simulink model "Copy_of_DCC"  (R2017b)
settings: Solver=FixedStepDiscrete  StartTime=0.0  StopTime=10.0  FixedStep=0.01  RelTol=1e-3  EnableMultiTasking=on
undefined symbols (not defined in the file): ASWTYPE_FALSE, ASWTYPE_TRUE, CbDCC_BMTMsgCmd_flg, CbDCC_BMVMsgCmd_flg, CbDCC_BSPMsgCmd_flg, CcDCC_BSTSendTi_ms, CcDCC_BulkSOC_pct, CcDCC_CCSTout_ms, CcDCC_CellTempFilterAvg_numb, CcDCC_ChrgCrnt0HysVolt_mV, CcDCC_ChrgFinOverTi_ms, CcDCC_ChrgMaxPackVoltLimt_V, CcDCC_ChrgSt2StepChrgTime_ms, CcDCC_ChrgStCutoffTime_ms, CcDCC_ChrgStFullChrgCrnt_A, CcDCC_CMLTout_ms, CcDCC_CommToutOverTi_ms, CcDCC_CRMAATout_ms, CcDCC_CRMCHMTout_ms, CcDCC_CRMTout_ms, CcDCC_CROAATout_ms, CcDCC_CROTout_ms, CcDCC_CSDTout_ms, CcDCC_CSTTout_ms, CcDCC_DC12VUnonnectTi_ms, CcDCC_DCChrgDispSOCPrmt_pct, CcDCC_DCChrgMismatch_ms, CcDCC_DCChrgPermitCfg_ms, CcDCC_DCChrgPrmtFltLvl_numb, CcDCC_DCChrgPrmtStop_ms, CcDCC_DCChrgStepCurr_A, CcDCC_DCChrgStop_ms, CcDCC_DCCrntUnctrolTi_ms, CcDCC_DCFullChrgHysVolt_mV, CcDCC_DCFullStepChrgTi1_ms, CcDCC_DCFullStepChrgTi2_ms, CcDCC_DCMaxChrgCurr_A, CcDCC_DCStepChrgWaitTime_ms, CcDCC_DCStop2DefaultTi_ms, CcDCC_DefaultWaitTi_ms, CcDCC_DiffDCChrgCrnt_A, CcDCC_DiffDCChrgCrntTi_ms, CcDCC_HeatChrgCrnt0Time_ms, CcDCC_HeatChrgCrnt1Time_ms, CcDCC_IsoDisableDelay_ms, CcDCC_MaxPackVoltLimt_V, CcDCC_SafeCur_A, CcDCC_StartChrgHysVolt_mV, CcDCC_StartDCChrgCellTemp_C, CcDCC_StepChrgCutoffTi_ms, CcDCC_StepChrgFullChrgCrnt_A, CcDCC_ToutDelay_ms, CcDCC_VehSpdFld_kmh, DCC_CONST0_NUMB, DCC_CONST1000_NUMB, DCC_CONST170_NUMB, DCC_RUNTIME_MS, Enum_BTMHeatReq, Enum_CTCCtrCtlConnMode, Enum_CTCCtrCtlState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
libraries: AIWAYS_Powertrain_BMS_lib x82
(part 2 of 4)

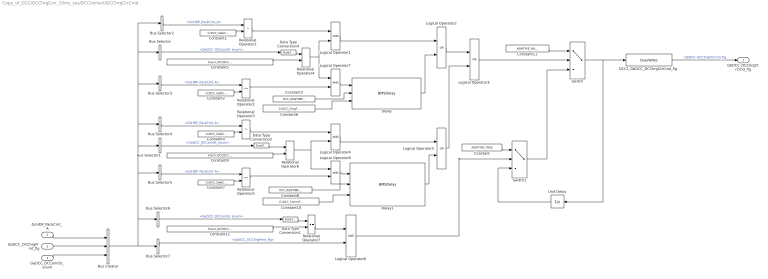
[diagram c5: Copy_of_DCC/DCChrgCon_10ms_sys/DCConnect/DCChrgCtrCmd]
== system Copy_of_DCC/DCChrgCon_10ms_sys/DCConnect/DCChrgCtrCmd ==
  GcHDP_PackCrnt_A : Inport
  GbDCC_DCChrgPrmt_flg : Inport  Port=2
  GeDCC_DCConnSt_enum : Inport  Port=3
  Bus Creator : BusCreator  Inputs=3
  Bus Selector : BusSelector  OutputSignals=GeDCC_DCConnSt_enum
  Bus Selector1 : BusSelector  OutputSignals=GeDCC_DCConnSt_enum
  Bus Selector{2..5} (4 alike) : BusSelector  OutputSignals=GcHDP_PackCrnt_A
  Bus Selector6 : BusSelector  OutputSignals=GeDCC_DCConnSt_enum
  Bus Selector7 : BusSelector  OutputSignals=GbDCC_DCChrgPrmt_flg
  Constant : Constant  Value=ASWTYPE_TRUE
  Constant{1..2,4,7} (4 alike) : Constant  Value=CcDCC_SafeCur_A
  Constant10 : Constant  Value=CcDCC_CommToutOverTi_ms
  Constant11 : Constant  Value=ASWTYPE_FALSE
  Constant12 : Constant  Value=Enum_DCCDCConnSt.Enum_DCCDCConnSt_CFG
  Constant3 : Constant  Value=DCC_RUNTIME_MS
  Constant5 : Constant  Value=Enum_DCCDCConnSt.Enum_DCCDCConnSt_ChrgFin
  Constant6 : Constant  Value=CcDCC_ChrgFinOverTi_ms
  Constant8 : Constant  Value=DCC_RUNTIME_MS
  Constant9 : Constant  Value=Enum_DCCDCConnSt.Enum_DCCDCConnSt_CommTout
  DCC1_GbDCC_DCChrgCtrCmd_flg : AIWAYS_Powertrain_BMS_lib/Signals/OverWrite  OverWrite_Value=CbDCC_DCChrgCtrCmdOvr_flg  OverWrite_flag=CbDCC_DCChrgCtrCmdOvrSwt_flg
  Data Type Conversion1 : DataTypeConversion
  Data Type Conversion2 : DataTypeConversion
  Data Type Conversion4 : DataTypeConversion
  Delay : AIWAYS_Powertrain_BMS_lib/Debounce & Delay/BMSDelay
  Delay1 : AIWAYS_Powertrain_BMS_lib/Debounce & Delay/BMSDelay
  Logical Operator{1,4,6..8} (5 alike) : Logic  AllPortsSameDT=off  OutDataTypeStr=boolean
  Logical Operator2 : Logic  Operator=OR  AllPortsSameDT=off  OutDataTypeStr=boolean
  Logical Operator3 : Logic  Operator=OR  AllPortsSameDT=off  OutDataTypeStr=boolean
  Logical Operator5 : Logic  Operator=OR  AllPortsSameDT=off  OutDataTypeStr=boolean
  Relational Operator1 : RelationalOperator  Operator=>  OutDataTypeStr=boolean
  Relational Operator2 : RelationalOperator  Operator=<=  OutDataTypeStr=boolean
  Relational Operator3 : RelationalOperator  Operator=>  OutDataTypeStr=boolean
  Relational Operator4 : RelationalOperator  Operator===  OutDataTypeStr=boolean
  Relational Operator5 : RelationalOperator  Operator=<=  OutDataTypeStr=boolean
  Relational Operator6 : RelationalOperator  Operator===  OutDataTypeStr=boolean
  Relational Operator7 : RelationalOperator  Operator===  OutDataTypeStr=boolean
  Switch : Switch  Criteria=u2 ~= 0
  Switch1 : Switch  Criteria=u2 ~= 0
  Unit Delay : UnitDelay  SampleTime=-1  StateName=StateName
  GbDCC_DCChrgCtrCmd_flg : Outport
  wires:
  Constant2/1 -> Relational Operator2/2
  Bus Selector7/1 -> Logical Operator6/2  "<GbDCC_DCChrgPrmt_flg>"
  Switch/1 -> DCC1_GbDCC_DCChrgCtrCmd_flg/1, Unit Delay/1
  Bus Selector6/1 -> Data Type Conversion1/1  "<GeDCC_DCConnSt_enum>"
  Constant12/1 -> Relational Operator7/2
  Relational Operator7/1 -> Logical Operator6/1
  Constant3/1 -> Delay/2
  Switch1/1 -> Switch/3
  Unit Delay/1 -> Switch1/3
  Logical Operator3/1 -> Switch/2
  Constant11/1 -> Switch/1
  Constant/1 -> Switch1/1
  Constant6/1 -> Delay/3
  Constant1/1 -> Relational Operator1/2
  Constant10/1 -> Delay1/3
  Constant7/1 -> Relational Operator5/2
  Constant9/1 -> Relational Operator6/2
  Constant4/1 -> Relational Operator3/2
  Constant8/1 -> Delay1/2
  Constant5/1 -> Relational Operator4/2
  Logical Operator6/1 -> Switch1/2
  Bus Selector2/1 -> Relational Operator1/1  "<GcHDP_PackCrnt_A>"
  Bus Selector/1 -> Data Type Conversion4/1  "<GeDCC_DCConnSt_enum>"
  Bus Selector1/1 -> Data Type Conversion2/1  "<GeDCC_DCConnSt_enum>"
  Bus Selector4/1 -> Relational Operator3/1  "<GcHDP_PackCrnt_A>"
  Bus Selector3/1 -> Relational Operator2/1  "<GcHDP_PackCrnt_A>"
  Bus Creator/1 -> Bus Selector2/1, Bus Selector/1, Bus Selector3/1, Bus Selector4/1, Bus Selector1/1, Bus Selector5/1, Bus Selector6/1, Bus Selector7/1
  Bus Selector5/1 -> Relational Operator5/1  "<GcHDP_PackCrnt_A>"
  DCC1_GbDCC_DCChrgCtrCmd_flg/1 -> GbDCC_DCChrgCtrCmd_flg/1  "GbDCC_DCChrgCtrCmd_flg"
  Data Type Conversion4/1 -> Relational Operator4/1
  Data Type Conversion2/1 -> Relational Operator6/1
  Data Type Conversion1/1 -> Relational Operator7/1
  Logical Operator1/1 -> Logical Operator2/1
  Relational Operator1/1 -> Logical Operator1/1
  Relational Operator4/1 -> Logical Operator7/1, Logical Operator1/2
  Relational Operator2/1 -> Logical Operator7/2
  Logical Operator7/1 -> Delay/1
  Delay/1 -> Logical Operator2/2
  Logical Operator2/1 -> Logical Operator3/1
  Logical Operator5/1 -> Logical Operator3/2
  Relational Operator6/1 -> Logical Operator8/1, Logical Operator4/2
  Relational Operator3/1 -> Logical Operator4/1
  Logical Operator4/1 -> Logical Operator5/1
  Relational Operator5/1 -> Logical Operator8/2
  Logical Operator8/1 -> Delay1/1
  Delay1/1 -> Logical Operator5/2
  GcHDP_PackCrnt_A/1 -> Bus Creator/1
  GbDCC_DCChrgPrmt_flg/1 -> Bus Creator/2
  GeDCC_DCConnSt_enum/1 -> Bus Creator/3

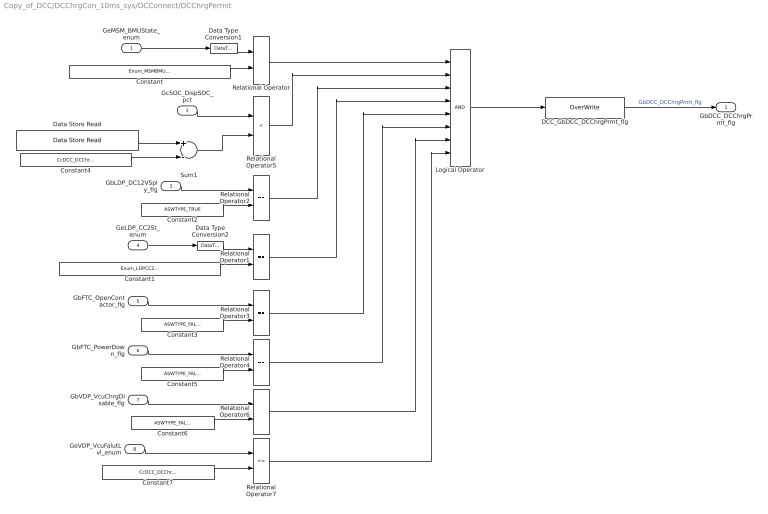
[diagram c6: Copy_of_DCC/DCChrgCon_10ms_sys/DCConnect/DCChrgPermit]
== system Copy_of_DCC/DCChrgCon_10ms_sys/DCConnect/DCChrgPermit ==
  GeMSM_BMUState_enum : Inport
  GcSOC_DispSOC_pct : Inport  Port=2
  GbLDP_DC12VSply_flg : Inport  Port=3
  GeLDP_CC2St_enum : Inport  Port=4
  GbFTC_OpenContactor_flg : Inport  Port=5
  GbFTC_PowerDown_flg : Inport  Port=6
  GbVDP_VcuChrgDisable_flg : Inport  Port=7
  GeVDP_VcuFalutLvl_enum : Inport  Port=8
  Constant : Constant  Value=Enum_MSMBMUState.Enum_MSMBMUState_Run
  Constant1 : Constant  Value=Enum_LDPCC2St.Enum_LDPCC2St_Connect
  Constant2 : Constant  Value=ASWTYPE_TRUE
  Constant3 : Constant  Value=ASWTYPE_FALSE
  Constant4 : Constant  Value=CcDCC_DCChrgDispSOCPrmt_pct
  Constant5 : Constant  Value=ASWTYPE_FALSE
  Constant6 : Constant  Value=ASWTYPE_FALSE
  Constant7 : Constant  Value=CcDCC_DCChrgPrmtFltLvl_numb
  DCC_GbDCC_DCChrgPrmt_flg : AIWAYS_Powertrain_BMS_lib/Signals/OverWrite  OverWrite_Value=CbDCC_DCChrgPrmtOvr_flg  OverWrite_flag=CbDCC_DCChrgPrmtOvrSwt_flg
  Data Store Read : AIWAYS_Powertrain_BMS_lib/Signals/Data Store Read  Priority=0  DSR=EcNVM_ChrgPermitMaxSOC_pct
  Data Type Conversion1 : DataTypeConversion
  Data Type Conversion2 : DataTypeConversion
  Logical Operator : Logic  Inputs=8  AllPortsSameDT=off  OutDataTypeStr=boolean
  Relational Operator{,1..4,6} (6 alike) : RelationalOperator  Operator===  OutDataTypeStr=boolean
  Relational Operator5 : RelationalOperator  Operator=<  OutDataTypeStr=boolean
  Relational Operator7 : RelationalOperator  Operator=<=  OutDataTypeStr=boolean
  Sum1 : Sum  Inputs=+-  OutDataTypeStr=Inherit: Inherit via back propagation  RndMeth=Zero
  GbDCC_DCChrgPrmt_flg : Outport
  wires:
  Constant/1 -> Relational Operator/2
  GeMSM_BMUState_enum/1 -> Data Type Conversion1/1
  Logical Operator/1 -> DCC_GbDCC_DCChrgPrmt_flg/1
  GbLDP_DC12VSply_flg/1 -> Relational Operator2/1
  GeLDP_CC2St_enum/1 -> Data Type Conversion2/1
  Constant1/1 -> Relational Operator1/2
  Data Type Conversion1/1 -> Relational Operator/1
  GcSOC_DispSOC_pct/1 -> Relational Operator5/1
  Constant2/1 -> Relational Operator2/2
  Relational Operator/1 -> Logical Operator/1
  DCC_GbDCC_DCChrgPrmt_flg/1 -> GbDCC_DCChrgPrmt_flg/1  "GbDCC_DCChrgPrmt_flg"
  Data Type Conversion2/1 -> Relational Operator1/1
  Relational Operator2/1 -> Logical Operator/3
  Relational Operator1/1 -> Logical Operator/4
  Constant3/1 -> Relational Operator3/2
  GbFTC_OpenContactor_flg/1 -> Relational Operator3/1
  Constant5/1 -> Relational Operator4/2
  GbFTC_PowerDown_flg/1 -> Relational Operator4/1
  Constant6/1 -> Relational Operator6/2
  GbVDP_VcuChrgDisable_flg/1 -> Relational Operator6/1
  Relational Operator3/1 -> Logical Operator/5
  Relational Operator4/1 -> Logical Operator/6
  Relational Operator6/1 -> Logical Operator/7
  GeVDP_VcuFalutLvl_enum/1 -> Relational Operator7/1
  Constant7/1 -> Relational Operator7/2
  Relational Operator7/1 -> Logical Operator/8
  Relational Operator5/1 -> Logical Operator/2
  Data Store Read/1 -> Sum1/1
  Constant4/1 -> Sum1/2
  Sum1/1 -> Relational Operator5/2

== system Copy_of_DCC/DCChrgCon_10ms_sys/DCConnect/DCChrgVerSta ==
  Constant2 : Constant  Value=ASWTYPE_TRUE
  DCC1_GbDCC_DCChrgVerSta_flg : AIWAYS_Powertrain_BMS_lib/Signals/OverWrite  OverWrite_Value=CbDCC_DCChrgVerStaOvr_flg  OverWrite_flag=CbDCC_DCChrgVerStaOvrSwt_flg
  GbDCC_DCChrgVerSta_flg : Outport
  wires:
  DCC1_GbDCC_DCChrgVerSta_flg/1 -> GbDCC_DCChrgVerSta_flg/1  "GbDCC_DCChrgVerSta_flg"
  Constant2/1 -> DCC1_GbDCC_DCChrgVerSta_flg/1

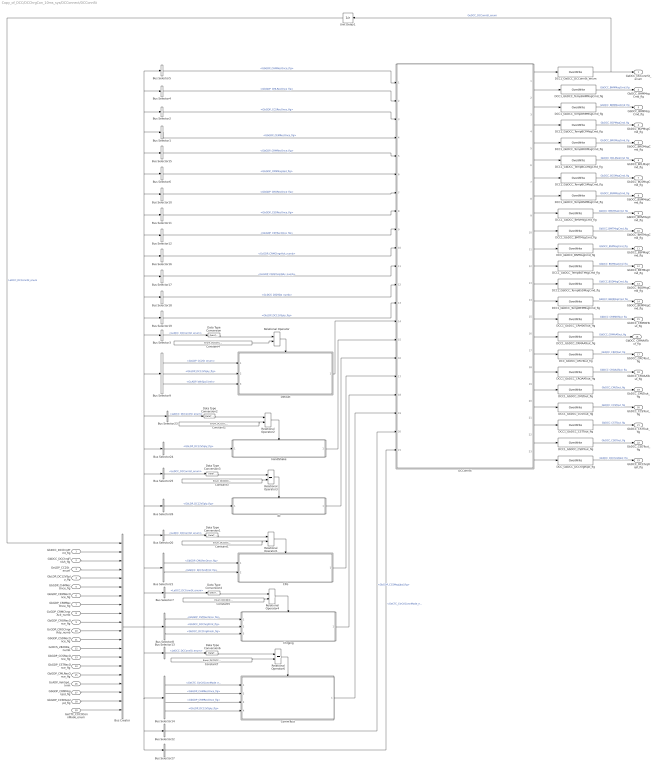
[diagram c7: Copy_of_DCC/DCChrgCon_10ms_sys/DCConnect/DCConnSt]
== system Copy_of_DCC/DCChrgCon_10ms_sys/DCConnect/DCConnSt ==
  GbDCC_DCChrgPrmt_flg : Inport
  GbDCC_DCChrgFinish_flg : Inport  Port=2
  GeLDP_CC2St_enum : Inport  Port=3
  GbLDP_DC12VSply_flg : Inport  Port=4
  GbGDP_CHMRecOnce_flg : Inport  Port=5
  GbGDP_CEMRecOnce_flg : Inport  Port=6
  GbGDP_CRMRecOnce_flg : Inport  Port=7
  GcGDP_CRMChrgrAck_numb : Inport  Port=8
  GbGDP_CRORecOnce_flg : Inport  Port=9
  GcGDP_CROChrgrRdy_numb : Inport  Port=10
  GbGDP_CSDRecOnce_flg : Inport  Port=11
  GcDCS_2829Da_numb : Inport  Port=12
  GbGDP_CCSRecOnce_flg : Inport  Port=13
  GbGDP_CSTRecOnce_flg : Inport  Port=14
  GbGDP_CMLRecOnce_flg : Inport  Port=15
  GcADP_VehSpd_kmh : Inport  Port=16
  GbGDP_CRMMsgUpd_flg : Inport  Port=17
  GbGDP_CCSMsgUpd_flg : Inport  Port=18
  GeCTC_CtrCtlConnMode_enum : Inport  Port=19
  Bus Creator : BusCreator  Inputs=20
  Bus Selector1 : BusSelector  OutputSignals=GbGDP_CEMRecOnce_flg
  Bus Selector10 : BusSelector  OutputSignals=GbGDP_CRORecOnce_flg
  Bus Selector11 : BusSelector  OutputSignals=GbGDP_CSDRecOnce_flg
  Bus Selector12 : BusSelector  OutputSignals=GbGDP_CSTRecOnce_flg
  Bus Selector{3,7,13,20,23,25} (6 alike) : BusSelector  OutputSignals=LeDCC_DCConnSt_enum
  Bus Selector14 : BusSelector  OutputSignals=GeCTC_CtrCtlConnMode_enum,GbGDP_CHMRecOnce_flg,GbGDP_CRMRecOnce_flg,GbLDP_DC12VSply_flg
  Bus Selector15 : BusSelector  OutputSignals=GbGDP_CRMRecOnce_flg
  Bus Selector16 : BusSelector  OutputSignals=GcGDP_CRMChrgrAck_numb
  Bus Selector17 : BusSelector  OutputSignals=GcGDP_CROChrgrRdy_numb
  Bus Selector18 : BusSelector  OutputSignals=GcDCS_2829Da_numb
  Bus Selector19 : BusSelector  OutputSignals=GbLDP_DC12VSply_flg
  Bus Selector2 : BusSelector  OutputSignals=GbGDP_CCSRecOnce_flg
  Bus Selector21 : BusSelector  OutputSignals=GbGDP_CMLRecOnce_flg,GbDCC_DCChrgPrmt_flg
  Bus Selector22 : BusSelector  OutputSignals=GbGDP_CCSMsgUpd_flg
  Bus Selector24 : BusSelector  OutputSignals=GbLDP_DC12VSply_flg
  Bus Selector26 : BusSelector  OutputSignals=GbLDP_DC12VSply_flg
  Bus Selector27 : BusSelector  OutputSignals=GeCTC_CtrCtlConnMode_enum
  Bus Selector4 : BusSelector  OutputSignals=GbGDP_CMLRecOnce_flg
  Bus Selector5 : BusSelector  OutputSignals=GbGDP_CHMRecOnce_flg
  Bus Selector6 : BusSelector  OutputSignals=GbGDP_CRMMsgUpd_flg
  Bus Selector8 : BusSelector  OutputSignals=GbGDP_CSTRecOnce_flg,GbDCC_DCChrgPrmt_flg,GbDCC_DCChrgFinish_flg
  Bus Selector9 : BusSelector  OutputSignals=GeLDP_CC2St_enum,GbLDP_DC12VSply_flg,GcADP_VehSpd_kmh
  CFG : Subsystem
  Chrging : Subsystem
  CommTout : Subsystem
  Constant1 : Constant  Value=Enum_DCCDCConnSt.Enum_DCCDCConnSt_CFG
  Constant2 : Constant  Value=Enum_DCCDCConnSt.Enum_DCCDCConnSt_HandShake
  Constant3 : Constant  Value=Enum_DCCDCConnSt.Enum_DCCDCConnSt_ID
  Constant4 : Constant  Value=Enum_DCCDCConnSt.Enum_DCCDCConnSt_Default
  Constant5 : Constant  Value=Enum_DCCDCConnSt.Enum_DCCDCConnSt_Chrging
  Constant7 : Constant  Value=Enum_DCCDCConnSt.Enum_DCCDCConnSt_CommTout
  DCC1_GbDCC_BMTMsgCmd_flg : AIWAYS_Powertrain_BMS_lib/Signals/OverWrite  OverWrite_Value=CbDCC_BMTMsgCmdOvr_flg  OverWrite_flag=CbDCC_BMTMsgCmdOvrSwt_flg
  DCC1_GbDCC_BMVMsgCmd_flg : AIWAYS_Powertrain_BMS_lib/Signals/OverWrite  OverWrite_Value=CbDCC_BMVMsgCmdOvr_flg  OverWrite_flag=CbDCC_BMVMsgCmdOvrSwt_flg
  DCC1_GbDCC_CCSTout_flg : AIWAYS_Powertrain_BMS_lib/Signals/OverWrite  OverWrite_Value=CbDCC_CCSToutOvr_flg  OverWrite_flag=CbDCC_CCSToutOvrSwt_flg
  DCC1_GbDCC_CMLTout_flg : AIWAYS_Powertrain_BMS_lib/Signals/OverWrite  OverWrite_Value=CbDCC_CMLToutOvr_flg  OverWrite_flag=CbDCC_CMLToutOvrSwt_flg
  DCC1_GbDCC_CRM00Tout_flg : AIWAYS_Powertrain_BMS_lib/Signals/OverWrite  OverWrite_Value=CbDCC_CRM00ToutOvr_flg  OverWrite_flag=CbDCC_CRM00ToutOvrSwt_flg
  DCC1_GbDCC_CRMAATout_flg : AIWAYS_Powertrain_BMS_lib/Signals/OverWrite  OverWrite_Value=CbDCC_CRMAAToutOvr_flg  OverWrite_flag=CbDCC_CRMAAToutOvrSwt_flg
  DCC1_GbDCC_CROAATout_flg : AIWAYS_Powertrain_BMS_lib/Signals/OverWrite  OverWrite_Value=CbDCC_CROAAToutOvr_flg  OverWrite_flag=CbDCC_CROAAToutOvrSwt_flg
  DCC1_GbDCC_CSDTout_flg : AIWAYS_Powertrain_BMS_lib/Signals/OverWrite  OverWrite_Value=CbDCC_CSDToutOvr_flg  OverWrite_flag=CbDCC_CSDToutOvrSwt_flg
  DCC1_GbDCC_CSTTout_flg : AIWAYS_Powertrain_BMS_lib/Signals/OverWrite  OverWrite_Value=CbDCC_CSTToutOvr_flg  OverWrite_flag=CbDCC_CSTToutOvrSwt_flg
  DCC1_GbDCC_TempBCLMsgCmd_flg : AIWAYS_Powertrain_BMS_lib/Signals/OverWrite  OverWrite_Value=CbDCC_BCLMsgCmdOvr_flg  OverWrite_flag=CbDCC_BCLMsgCmdOvrSwt_flg
  DCC1_GbDCC_TempBCPMsgCmd_flg : AIWAYS_Powertrain_BMS_lib/Signals/OverWrite  OverWrite_Value=CbDCC_BCPMsgCmdOvr_flg  OverWrite_flag=CbDCC_BCPMsgCmdOvrSwt_flg
  DCC1_GbDCC_TempBCSMsgCmd_flg : AIWAYS_Powertrain_BMS_lib/Signals/OverWrite  OverWrite_Value=CbDCC_BCSMsgCmdOvr_flg  OverWrite_flag=CbDCC_BCSMsgCmdOvrSwt_flg
  DCC1_GbDCC_TempBEMMsgCmd_flg : AIWAYS_Powertrain_BMS_lib/Signals/OverWrite  OverWrite_Value=CbDCC_BEMMsgCmdOvr_flg  OverWrite_flag=CbDCC_BEMMsgCmdOvrSwt_flg
  DCC1_GbDCC_TempBHMMsgCmd_flg : AIWAYS_Powertrain_BMS_lib/Signals/OverWrite  OverWrite_Value=CbDCC_BHMMsgCmdOvr_flg  OverWrite_flag=CbDCC_BHMMsgCmdOvrSwt_flg
  DCC1_GbDCC_TempBRMMsgCmd_flg : AIWAYS_Powertrain_BMS_lib/Signals/OverWrite  OverWrite_Value=CbDCC_BRMMsgCmdOvr_flg  OverWrite_flag=CbDCC_BRMMsgCmdOvrSwt_flg
  DCC1_GbDCC_TempBROMsgCmd_flg : AIWAYS_Powertrain_BMS_lib/Signals/OverWrite  OverWrite_Value=CbDCC_BROMsgCmdOvr_flg  OverWrite_flag=CbDCC_BROMsgCmdOvrSwt_flg
  DCC1_GbDCC_TempBSDMsgCmd_flg : AIWAYS_Powertrain_BMS_lib/Signals/OverWrite  OverWrite_Value=CbDCC_BSDMsgCmdOvr_flg  OverWrite_flag=CbDCC_BSDMsgCmdOvrSwt_flg
  DCC1_GbDCC_TempBSMMsgCmd_flg : AIWAYS_Powertrain_BMS_lib/Signals/OverWrite  OverWrite_Value=CbDCC_BSMMsgCmdOvr_flg  OverWrite_flag=CbDCC_BSMMsgCmdOvrSwt_flg
  DCC1_GbDCC_TempBSTMsgCmd_flg : AIWAYS_Powertrain_BMS_lib/Signals/OverWrite  OverWrite_Value=CbDCC_BSTMsgCmdOvr_flg  OverWrite_flag=CbDCC_BSTMsgCmdOvrSwt_flg
  DCC1_GeDCC_DCConnSt_enum : AIWAYS_Powertrain_BMS_lib/Signals/OverWrite  OverWrite_Value=CeDCC_DCConnStOvr_enum  OverWrite_flag=CbDCC_DCConnStOvrSwt_flg
  DCC_GbDCC_BSPMsgCmd_flg : AIWAYS_Powertrain_BMS_lib/Signals/OverWrite  OverWrite_Value=CbDCC_BSPMsgCmdOvr_flg  OverWrite_flag=CbDCC_BSPMsgCmdOvrSwt_flg
  DCC_GbDCC_CROTout_flg : AIWAYS_Powertrain_BMS_lib/Signals/OverWrite  OverWrite_Value=CbDCC_CROToutOvr_flg  OverWrite_flag=CbDCC_CROToutOvrSwt_flg
  DCC_GbDCC_DCChrgRqst_flg : AIWAYS_Powertrain_BMS_lib/Signals/OverWrite  OverWrite_Value=CbDCC_DCChrgRqstOvr_flg  OverWrite_flag=CbDCC_DCChrgRqstOvrSwt_flg
  DCConnSt : Stateflow chart  TreatAsAtomicUnit=on
  Data Type Conversion{,1..4,6} (6 alike) : DataTypeConversion
  Default : Subsystem
  HandShake : Subsystem
  ID : Subsystem
  Relational Operator{,1..4,6} (6 alike) : RelationalOperator  Operator===  OutDataTypeStr=boolean
  Unit Delay1 : UnitDelay  SampleTime=-1  StateName=StateName
  GeDCC_DCConnSt_enum : Outport
  GbDCC_BHMMsgCmd_flg : Outport  Port=2
  GbDCC_BRMMsgCmd_flg : Outport  Port=3
  GbDCC_BCPMsgCmd_flg : Outport  Port=4
  GbDCC_BROMsgCmd_flg : Outport  Port=5
  GbDCC_BCLMsgCmd_flg : Outport  Port=6
  GbDCC_BCSMsgCmd_flg : Outport  Port=7
  GbDCC_BSMMsgCmd_flg : Outport  Port=8
  GbDCC_BMVMsgCmd_flg : Outport  Port=9
  GbDCC_BMTMsgCmd_flg : Outport  Port=10
  GbDCC_BSPMsgCmd_flg : Outport  Port=11
  GbDCC_BSTMsgCmd_flg : Outport  Port=12
  GbDCC_BSDMsgCmd_flg : Outport  Port=13
  GbDCC_BEMMsgCmd_flg : Outport  Port=14
  GbDCC_CRM00Tout_flg : Outport  Port=15
  GbDCC_CRMAATout_flg : Outport  Port=16
  GbDCC_CROTout_flg : Outport  Port=17
  GbDCC_CROAATout_flg : Outport  Port=18
  GbDCC_CMLTout_flg : Outport  Port=19
  GbDCC_CCSTout_flg : Outport  Port=20
  GbDCC_CSTTout_flg : Outport  Port=21
  GbDCC_CSDTout_flg : Outport  Port=22
  GbDCC_DCChrgRqst_flg : Outport  Port=23
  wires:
  Bus Selector19/1 -> DCConnSt/13(GbLDP_DC12VSply_flg)  "<GbLDP_DC12VSply_flg>"
  Bus Selector18/1 -> DCConnSt/12(GcDCS_2829Da_numb)  "<GcDCS_2829Da_numb>"
  Bus Selector17/1 -> DCConnSt/11(GcGDP_CROChrgrRdy_numb)  "<GcGDP_CROChrgrRdy_numb>"
  Bus Selector16/1 -> DCConnSt/10(GcGDP_CRMChrgrAck_numb)  "<GcGDP_CRMChrgrAck_numb>"
  Bus Selector12/1 -> DCConnSt/9(GbGDP_CSTRecOnce_flg)  "<GbGDP_CSTRecOnce_flg>"
  Bus Selector11/1 -> DCConnSt/8(GbGDP_CSDRecOnce_flg)  "<GbGDP_CSDRecOnce_flg>"
  Bus Selector10/1 -> DCConnSt/7(GbGDP_CRORecOnce_flg)  "<GbGDP_CRORecOnce_flg>"
  Bus Selector6/1 -> DCConnSt/6(GbGDP_CRMMsgUpd_flg)  "<GbGDP_CRMMsgUpd_flg>"
  Bus Selector5/1 -> DCConnSt/1(GbGDP_CHMRecOnce_flg)  "<GbGDP_CHMRecOnce_flg>"
  Bus Selector4/1 -> DCConnSt/2(GbGDP_CMLRecOnce_flg)  "<GbGDP_CMLRecOnce_flg>"
  Bus Selector2/1 -> DCConnSt/3(GbGDP_CCSRecOnce_flg)  "<GbGDP_CCSRecOnce_flg>"
  Bus Selector1/1 -> DCConnSt/4(GbGDP_CEMRecOnce_flg)  "<GbGDP_CEMRecOnce_flg>"
  DCConnSt/22(GbDCC_CSDTout_flg) -> DCC1_GbDCC_CSDTout_flg/1
  DCConnSt/21(GbDCC_CSTTout_flg) -> DCC1_GbDCC_CSTTout_flg/1
  DCConnSt/20(GbDCC_CCSTout_flg) -> DCC1_GbDCC_CCSTout_flg/1
  DCConnSt/19(GbDCC_CMLTout_flg) -> DCC1_GbDCC_CMLTout_flg/1
  DCConnSt/18(GbDCC_CROAATout_flg) -> DCC1_GbDCC_CROAATout_flg/1
  DCConnSt/17(GbDCC_CROTout_flg) -> DCC_GbDCC_CROTout_flg/1
  DCConnSt/16(GbDCC_CRMAATout_flg) -> DCC1_GbDCC_CRMAATout_flg/1
  DCC1_GbDCC_CSDTout_flg/1 -> GbDCC_CSDTout_flg/1  "GbDCC_CSDTout_flg"
  DCC1_GbDCC_CSTTout_flg/1 -> GbDCC_CSTTout_flg/1  "GbDCC_CSTTout_flg"
  DCC1_GbDCC_CCSTout_flg/1 -> GbDCC_CCSTout_flg/1  "GbDCC_CCSTout_flg"
  DCC_GbDCC_CROTout_flg/1 -> GbDCC_CROTout_flg/1  "GbDCC_CROTout_flg"
  DCC1_GbDCC_CROAATout_flg/1 -> GbDCC_CROAATout_flg/1  "GbDCC_CROAATout_flg"
  DCC1_GbDCC_CMLTout_flg/1 -> GbDCC_CMLTout_flg/1  "GbDCC_CMLTout_flg"
  DCC1_GbDCC_CRMAATout_flg/1 -> GbDCC_CRMAATout_flg/1  "GbDCC_CRMAATout_flg"
  DCC1_GbDCC_CRM00Tout_flg/1 -> GbDCC_CRM00Tout_flg/1  "GbDCC_CRM00Tout_flg"
  DCConnSt/15(GbDCC_CRM00Tout_flg) -> DCC1_GbDCC_CRM00Tout_flg/1
  Bus Selector15/1 -> DCConnSt/5(GbGDP_CRMRecOnce_flg)  "<GbGDP_CRMRecOnce_flg>"
  Unit Delay1/1 -> Bus Creator/1  "LeDCC_DCConnSt_enum"
  Data Type Conversion6/1 -> Relational Operator6/1
  Data Type Conversion4/1 -> Relational Operator4/1
  Data Type Conversion/1 -> Relational Operator/1
  DCConnSt/1(GeDCC_DCConnSt_enum) -> DCC1_GeDCC_DCConnSt_enum/1
  Bus Selector9/3 -> Default/3(GcADP_VehSpd_kmh)  "<GcADP_VehSpd_kmh>"
  Chrging/1(LbDCC_DCChrging2ChrgFin_flg) -> DCConnSt/18(LbDCC_DCChrging2ChrgFin_flg)
  CommTout/1(LbDCC_DCCommTout2Default_flg) -> DCConnSt/19(LbDCC_DCCommTout2Default_flg)
  Default/1(LbDCC_DCDefault2Handshake_flg) -> DCConnSt/14(LbDCC_DCDefault2Handshake_flg)
  DCC1_GbDCC_BMVMsgCmd_flg/1 -> GbDCC_BMVMsgCmd_flg/1  "GbDCC_BMVMsgCmd_flg"
  DCC1_GbDCC_BMTMsgCmd_flg/1 -> GbDCC_BMTMsgCmd_flg/1  "GbDCC_BMTMsgCmd_flg"
  DCC_GbDCC_BSPMsgCmd_flg/1 -> GbDCC_BSPMsgCmd_flg/1  "GbDCC_BSPMsgCmd_flg"
  DCC1_GeDCC_DCConnSt_enum/1 -> GeDCC_DCConnSt_enum/1, Unit Delay1/1  "GeDCC_DCConnSt_enum"
  Bus Selector14/1 -> CommTout/1(GeCTC_CtrCtlConnMode_enum)  "<GeCTC_CtrCtlConnMode_enum>"
  Bus Selector13/1 -> Data Type Conversion6/1  "<LeDCC_DCConnSt_enum>"
  Bus Selector8/3 -> Chrging/3(GbDCC_DCChrgFinish_flg)  "<GbDCC_DCChrgFinish_flg>"
  Bus Selector8/2 -> Chrging/2(GbDCC_DCChrgPrmt_flg)  "<GbDCC_DCChrgPrmt_flg>"
  Bus Selector8/1 -> Chrging/1(GbGDP_CSTRecOnce_flg)  "<GbGDP_CSTRecOnce_flg>"
  Bus Selector9/2 -> Default/2(GbLDP_DC12VSply_flg)  "<GbLDP_DC12VSply_flg>"
  Bus Selector9/1 -> Default/1(GeLDP_CC2St_enum)  "<GeLDP_CC2St_enum>"
  Bus Selector7/1 -> Data Type Conversion4/1  "<LeDCC_DCConnSt_enum>"
  Bus Selector3/1 -> Data Type Conversion/1  "<LeDCC_DCConnSt_enum>"
  Relational Operator6/1 -> CommTout/Enable
  Constant7/1 -> Relational Operator6/2
  Relational Operator4/1 -> Chrging/Enable
  Constant5/1 -> Relational Operator4/2
  Constant4/1 -> Relational Operator/2
  Relational Operator/1 -> Default/Enable
  Data Type Conversion1/1 -> Relational Operator1/1
  CFG/1(LbDCC_DCCFG2ChrgFinish_flg) -> DCConnSt/17(LbDCC_DCCFG2ChrgFinish_flg)
  Bus Selector21/2 -> CFG/2(GbDCC_DCChrgPrmt_flg)  "<GbDCC_DCChrgPrmt_flg>"
  Bus Selector21/1 -> CFG/1(GbGDP_CMLRecOnce_flg)  "<GbGDP_CMLRecOnce_flg>"
  Bus Selector20/1 -> Data Type Conversion1/1  "<LeDCC_DCConnSt_enum>"
  Relational Operator1/1 -> CFG/Enable
  Constant1/1 -> Relational Operator1/2
  Bus Selector22/1 -> DCConnSt/20(GbGDP_CCSMsgUpd_flg)  "<GbGDP_CCSMsgUpd_flg>"
  Data Type Conversion2/1 -> Relational Operator2/1
  Bus Selector23/1 -> Data Type Conversion2/1  "<LeDCC_DCConnSt_enum>"
  Relational Operator2/1 -> HandShake/Enable
  Constant2/1 -> Relational Operator2/2
  Bus Selector24/1 -> HandShake/1(GbLDP_DC12VSply_flg)  "<GbLDP_DC12VSply_flg>"
  Data Type Conversion3/1 -> Relational Operator3/1
  Bus Selector25/1 -> Data Type Conversion3/1  "<LeDCC_DCConnSt_enum>"
  Relational Operator3/1 -> ID/Enable
  Constant3/1 -> Relational Operator3/2
  Bus Selector26/1 -> ID/1(GbLDP_DC12VSply_flg)  "<GbLDP_DC12VSply_flg>"
  Bus Creator/1 -> Bus Selector26/1, Bus Selector25/1, Bus Selector24/1, Bus Selector23/1, Bus Selector3/1, Bus Selector11/1, Bus Selector15/1, Bus Selector1/1, Bus Selector2/1, Bus Selector4/1, Bus Selector5/1, Bus Selector6/1, Bus Selector10/1, Bus Selector12/1, Bus Selector16/1, Bus Selector17/1, Bus Selector18/1, Bus Selector19/1, Bus Selector9/1, Bus Selector20/1, Bus Selector21/1, Bus Selector7/1, Bus Selector8/1, Bus Selector13/1, Bus Selector27/1, Bus Selector22/1, Bus Selector14/1
  HandShake/1(LbDCC_DCHandShake2Default_flg) -> DCConnSt/15(LbDCC_DCHandShake2Default_flg)
  ID/1(LbDCC_DCID2Default_flg) -> DCConnSt/16(LbDCC_DCID2Default_flg)
  Bus Selector14/2 -> CommTout/2(GbGDP_CHMRecOnce_flg)  "<GbGDP_CHMRecOnce_flg>"
  Bus Selector14/3 -> CommTout/3(GbGDP_CRMRecOnce_flg)  "<GbGDP_CRMRecOnce_flg>"
  Bus Selector14/4 -> CommTout/4(GbLDP_DC12VSply_flg)  "<GbLDP_DC12VSply_flg>"
  DCConnSt/9(GbDCC_BMVMsgCmd_flg) -> DCC1_GbDCC_BMVMsgCmd_flg/1
  DCConnSt/10(GbDCC_BMTMsgCmd_flg) -> DCC1_GbDCC_BMTMsgCmd_flg/1
  DCConnSt/11(GbDCC_BSPMsgCmd_flg) -> DCC_GbDCC_BSPMsgCmd_flg/1
  DCConnSt/8(GbDCC_BSMMsgCmd_flg) -> DCC1_GbDCC_TempBSMMsgCmd_flg/1
  DCConnSt/2(GbDCC_BHMMsgCmd_flg) -> DCC1_GbDCC_TempBHMMsgCmd_flg/1
  DCConnSt/4(GbDCC_BCPMsgCmd_flg) -> DCC1_GbDCC_TempBCPMsgCmd_flg/1
  DCConnSt/6(GbDCC_BCLMsgCmd_flg) -> DCC1_GbDCC_TempBCLMsgCmd_flg/1
  DCConnSt/3(GbDCC_BRMMsgCmd_flg) -> DCC1_GbDCC_TempBRMMsgCmd_flg/1
  DCConnSt/7(GbDCC_BCSMsgCmd_flg) -> DCC1_GbDCC_TempBCSMsgCmd_flg/1
  DCConnSt/13(GbDCC_BSDMsgCmd_flg) -> DCC1_GbDCC_TempBSDMsgCmd_flg/1
  DCConnSt/14(GbDCC_BEMMsgCmd_flg) -> DCC1_GbDCC_TempBEMMsgCmd_flg/1
  DCConnSt/12(GbDCC_BSTMsgCmd_flg) -> DCC1_GbDCC_TempBSTMsgCmd_flg/1
  DCConnSt/5(GbDCC_BROMsgCmd_flg) -> DCC1_GbDCC_TempBROMsgCmd_flg/1
  DCC1_GbDCC_TempBHMMsgCmd_flg/1 -> GbDCC_BHMMsgCmd_flg/1  "GbDCC_BHMMsgCmd_flg"
  DCC1_GbDCC_TempBRMMsgCmd_flg/1 -> GbDCC_BRMMsgCmd_flg/1  "GbDCC_BRMMsgCmd_flg"
  DCC1_GbDCC_TempBCPMsgCmd_flg/1 -> GbDCC_BCPMsgCmd_flg/1  "GbDCC_BCPMsgCmd_flg"
  DCC1_GbDCC_TempBROMsgCmd_flg/1 -> GbDCC_BROMsgCmd_flg/1  "GbDCC_BROMsgCmd_flg"
  DCC1_GbDCC_TempBCLMsgCmd_flg/1 -> GbDCC_BCLMsgCmd_flg/1  "GbDCC_BCLMsgCmd_flg"
  DCC1_GbDCC_TempBCSMsgCmd_flg/1 -> GbDCC_BCSMsgCmd_flg/1  "GbDCC_BCSMsgCmd_flg"
  DCC1_GbDCC_TempBSMMsgCmd_flg/1 -> GbDCC_BSMMsgCmd_flg/1  "GbDCC_BSMMsgCmd_flg"
  DCC1_GbDCC_TempBEMMsgCmd_flg/1 -> GbDCC_BEMMsgCmd_flg/1  "GbDCC_BEMMsgCmd_flg"
  DCC1_GbDCC_TempBSTMsgCmd_flg/1 -> GbDCC_BSTMsgCmd_flg/1  "GbDCC_BSTMsgCmd_flg"
  DCC1_GbDCC_TempBSDMsgCmd_flg/1 -> GbDCC_BSDMsgCmd_flg/1  "GbDCC_BSDMsgCmd_flg"
  GbDCC_DCChrgPrmt_flg/1 -> Bus Creator/2
  GbDCC_DCChrgFinish_flg/1 -> Bus Creator/3
  GeLDP_CC2St_enum/1 -> Bus Creator/4
  GbLDP_DC12VSply_flg/1 -> Bus Creator/5
  GbGDP_CHMRecOnce_flg/1 -> Bus Creator/6
  GbGDP_CEMRecOnce_flg/1 -> Bus Creator/7
  GbGDP_CRMRecOnce_flg/1 -> Bus Creator/8
  GcGDP_CRMChrgrAck_numb/1 -> Bus Creator/9
  GbGDP_CRORecOnce_flg/1 -> Bus Creator/10
  GcGDP_CROChrgrRdy_numb/1 -> Bus Creator/11
  GbGDP_CSDRecOnce_flg/1 -> Bus Creator/12
  GcDCS_2829Da_numb/1 -> Bus Creator/13
  GbGDP_CCSRecOnce_flg/1 -> Bus Creator/14
  GbGDP_CSTRecOnce_flg/1 -> Bus Creator/15
  GbGDP_CMLRecOnce_flg/1 -> Bus Creator/16
  GcADP_VehSpd_kmh/1 -> Bus Creator/17
  GbGDP_CRMMsgUpd_flg/1 -> Bus Creator/18
  GbGDP_CCSMsgUpd_flg/1 -> Bus Creator/19
  GeCTC_CtrCtlConnMode_enum/1 -> Bus Creator/20
  Bus Selector27/1 -> DCConnSt/21(GeCTC_CtrCtlConnMode_enum)  "<GeCTC_CtrCtlConnMode_enum>"
  DCC_GbDCC_DCChrgRqst_flg/1 -> GbDCC_DCChrgRqst_flg/1  "GbDCC_DCChrgRqst_flg"
  DCConnSt/23(GbDCC_DCChrgRqst_flg) -> DCC_GbDCC_DCChrgRqst_flg/1

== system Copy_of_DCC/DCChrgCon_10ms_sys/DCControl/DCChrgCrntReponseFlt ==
  GcGDP_CCSCurOut_A : Inport
  GbGDP_CCSRecOnce_flg : Inport  Port=2
  GeDCC_DCChrgState_enum : Inport  Port=3
  GcDCC_DCChrgCrntRqst_A : Inport  Port=4
  BMSDebounceStartZero : AIWAYS_Powertrain_BMS_lib/Debounce & Delay/BMSDebounceStartZero
  Constant1 : Constant  Value=CcDCC_DiffDCChrgCrnt_A
  Constant2 : Constant  Value=Enum_DCCDCChrgState.Enum_DCCDCChrgState_Chrg
  Constant3 : Constant  Value=Enum_DCCDCChrgState.Enum_DCCDCChrgState_StepChrg
  Constant4 : Constant  Value=CcDCC_DiffDCChrgCrntTi_ms
  Constant5 : Constant  Value=DCC_RUNTIME_MS
  Constant6 : Constant  Value=CcDCC_DiffDCChrgCrntTi_ms
  Constant7 : Constant  Value=DCC_RUNTIME_MS
  Constant8 : Constant  Value=ASWTYPE_TRUE
  DCC_GbDCC_DCChrgCrntFlt_flg : AIWAYS_Powertrain_BMS_lib/Signals/OverWrite  OverWrite_Value=CbDCC_DCChrgCrntFltOvr_flg  OverWrite_flag=CbDCC_DCChrgCrntFltOvrSwt_flg
  Data Type Conversion3 : DataTypeConversion
  DiffValue : AIWAYS_Powertrain_BMS_lib/Mathematical Functions/DiffValue
  Logical Operator : Logic  Operator=OR  AllPortsSameDT=off  OutDataTypeStr=boolean
  Logical Operator1 : Logic  Inputs=3  AllPortsSameDT=off  OutDataTypeStr=boolean
  Relational Operator1 : RelationalOperator  Operator=>  OutDataTypeStr=boolean
  Relational Operator2 : RelationalOperator  Operator===  OutDataTypeStr=boolean
  Relational Operator3 : RelationalOperator  Operator===  OutDataTypeStr=boolean
  Relational Operator4 : RelationalOperator  Operator===  OutDataTypeStr=boolean
  GbDCC_DCChrgCrntFlt_flg : Outport
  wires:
  Data Type Conversion3/1 -> Relational Operator3/1, Relational Operator2/1
  Relational Operator1/1 -> Logical Operator1/2
  Logical Operator/1 -> Logical Operator1/1
  Relational Operator3/1 -> Logical Operator/2
  Relational Operator2/1 -> Logical Operator/1
  Constant3/1 -> Relational Operator3/2
  GeDCC_DCChrgState_enum/1 -> Data Type Conversion3/1
  Constant2/1 -> Relational Operator2/2
  Constant1/1 -> Relational Operator1/2
  GcDCC_DCChrgCrntRqst_A/1 -> DiffValue/1
  GcGDP_CCSCurOut_A/1 -> DiffValue/2
  DiffValue/1 -> Relational Operator1/1
  Logical Operator1/1 -> BMSDebounceStartZero/1
  Constant4/1 -> BMSDebounceStartZero/2
  Constant6/1 -> BMSDebounceStartZero/4
  Constant5/1 -> BMSDebounceStartZero/3
  Constant7/1 -> BMSDebounceStartZero/5
  BMSDebounceStartZero/1 -> DCC_GbDCC_DCChrgCrntFlt_flg/1
  Constant8/1 -> Relational Operator4/2
  GbGDP_CCSRecOnce_flg/1 -> Relational Operator4/1
  Relational Operator4/1 -> Logical Operator1/3
  DCC_GbDCC_DCChrgCrntFlt_flg/1 -> GbDCC_DCChrgCrntFlt_flg/1  "GbDCC_DCChrgCrntFlt_flg"

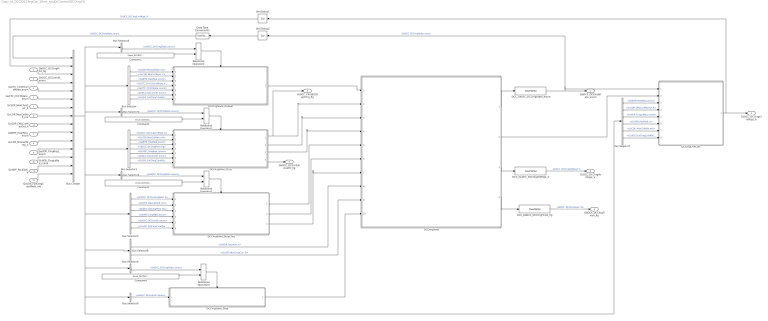
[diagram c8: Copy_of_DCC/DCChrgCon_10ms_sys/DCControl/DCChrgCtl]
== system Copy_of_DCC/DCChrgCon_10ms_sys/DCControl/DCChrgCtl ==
  GbDCC_DCChrgPrmt_flg : Inport
  GeDCC_DCConnSt_enum : Inport  Port=2
  GeCTC_CtrCtlConnMode_enum : Inport  Port=3
  GeCTC_CtrCtlState_enum : Inport  Port=4
  GcSOP_MaxChrgCurr_A : Inport  Port=5
  GcCDP_MaxCellVolt_mV : Inport  Port=6
  GeBTM_HeatReq_enum : Inport  Port=7
  GcCDP_MinCellTemp_C : Inport  Port=8
  GeVDP_ChrgRqst_enum : Inport  Port=9
  GcVDP_ChrgLdReq_numb : Inport  Port=10
  GcHDP_PackVolt_V : Inport  Port=11
  GcUDS_FullChrgCutoffVolt_mV : Inport  Port=12
  GcGDP_CMLCurMaxOut_A : Inport  Port=13
  Bus Creator : BusCreator  Inputs=15
  Bus Selector : BusSelector  OutputSignals=GcCDP_MaxCellVolt_mV,GcCDP_MinCellTemp_C,GeBTM_HeatReq_enum,GeCTC_CtrCtlConnMode_enum,GeCTC_CtrCtlState_enum,GeDCC_DCConnSt_enum,GcUDS_FullChrgCutoffVolt_mV
  Bus Selector1 : BusSelector  OutputSignals=GcDCC_DCChrgCrntRqst_A,GcCDP_MaxCellVolt_mV,GeBTM_HeatReq_enum,GbDCC_DCChrgPrmt_flg,GeVDP_ChrgRqst_enum,GeDCC_DCConnSt_enum,GcUDS_FullChrgCutoffVolt_mV
  Bus Selector{2,4..6} (4 alike) : BusSelector  OutputSignals=GeDCC_DCChrgState_enum
  Bus Selector3 : BusSelector  OutputSignals=GcDCC_DCChrgCrntRqst_A,GcCDP_MaxCellVolt_mV,GbDCC_DCChrgPrmt_flg,GeVDP_ChrgRqst_enum,GeDCC_DCConnSt_enum,GcUDS_FullChrgCutoffVolt_mV
  Bus Selector7 : BusSelector  OutputSignals=GeBTM_HeatReq_enum,GcGDP_CMLCurMaxOut_A,GcVDP_ChrgLdReq_numb,GcHDP_PackVolt_V,GcCDP_MaxCellVolt_mV,GcUDS_FullChrgCutoffVolt_mV
  Bus Selector8 : BusSelector  OutputSignals=GcHDP_PackVolt_V,GcSOP_MaxChrgCurr_A
  Bus Selector9 : BusSelector  OutputSignals=GeDCC_DCConnSt_enum
  Constant1 : Constant  Value=Enum_DCCDCChrgState.Enum_DCCDCChrgState_Chrg
  Constant2 : Constant  Value=Enum_DCCDCChrgState.Enum_DCCDCChrgState_Default
  Constant3 : Constant  Value=Enum_DCCDCChrgState.Enum_DCCDCChrgState_StepChrg
  Constant4 : Constant  Value=Enum_DCCDCChrgState.Enum_DCCDCChrgState_Stop
  DCC_GbDCC_DCChrgFinish_flg : AIWAYS_Powertrain_BMS_lib/Signals/OverWrite  OverWrite_Value=CbDCC_DCChrgFinishOvr_flg  OverWrite_flag=CbDCC_DCChrgFinishOvrSwt_flg
  DCC_GcDCC_DCChrgVoltRqst_V : AIWAYS_Powertrain_BMS_lib/Signals/OverWrite  OverWrite_Value=CcDCC_DCChrgVoltRqstOvr_V  OverWrite_flag=CbDCC_DCChrgVoltRqstOvrSwt_flg
  DCC_GeDCC_DCChrgState_enum : AIWAYS_Powertrain_BMS_lib/Signals/OverWrite  OverWrite_Value=CeDCC_DCChrgStateOvr_enum  OverWrite_flag=CbDCC_DCChrgStateOvrSwt_flg
  DCChrgCrntCalc : Subsystem
  DCChrgState : Stateflow chart  TreatAsAtomicUnit=on
  DCChrgState_Chrg : Subsystem
  DCChrgState_Default : Subsystem
  DCChrgState_StepChrg : Subsystem
  DCChrgState_Stop : Subsystem
  Data Type Conversion1 : DataTypeConversion
  Relational Operator{1..4} (4 alike) : RelationalOperator  Operator===  OutDataTypeStr=boolean
  Unit Delay1 : UnitDelay  SampleTime=-1  StateName=StateName
  Unit Delay2 : UnitDelay  SampleTime=-1  StateName=StateName
  GeDCC_DCChrgState_enum : Outport
  GcDCC_DCChrgCrntRqst_A : Outport  Port=2
  GcDCC_DCChrgVoltRqst_V : Outport  Port=3
  GbDCC_DCChrgFinish_flg : Outport  Port=4
  GbDCC_DCCrntUnctrolFlt_flg : Outport  Port=5
  LbDCC_ChrgSt2StepChrg_flg : Outport  Port=6
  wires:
  GeCTC_CtrCtlConnMode_enum/1 -> Bus Creator/5
  GeCTC_CtrCtlState_enum/1 -> Bus Creator/6
  GcSOP_MaxChrgCurr_A/1 -> Bus Creator/7
  GcCDP_MaxCellVolt_mV/1 -> Bus Creator/8
  GcGDP_CMLCurMaxOut_A/1 -> Bus Creator/9
  GeBTM_HeatReq_enum/1 -> Bus Creator/10
  GcCDP_MinCellTemp_C/1 -> Bus Creator/11
  GeVDP_ChrgRqst_enum/1 -> Bus Creator/12
  GcVDP_ChrgLdReq_numb/1 -> Bus Creator/13
  GcHDP_PackVolt_V/1 -> Bus Creator/14
  GeDCC_DCConnSt_enum/1 -> Bus Creator/4
  GbDCC_DCChrgPrmt_flg/1 -> Bus Creator/3
  Bus Selector/1 -> DCChrgState_Default/1(GcCDP_MaxCellVolt_mV)  "<GcCDP_MaxCellVolt_mV>"
  Bus Selector/2 -> DCChrgState_Default/2(GcCDP_MinCellTemp_C)  "<GcCDP_MinCellTemp_C>"
  Bus Selector/3 -> DCChrgState_Default/3(GeBTM_HeatReq_enum)  "<GeBTM_HeatReq_enum>"
  Bus Selector/4 -> DCChrgState_Default/4(GeCTC_CtrCtlConnMode_enum)  "<GeCTC_CtrCtlConnMode_enum>"
  Bus Selector/5 -> DCChrgState_Default/5(GeCTC_CtrCtlState_enum)  "<GeCTC_CtrCtlState_enum>"
  Bus Selector/6 -> DCChrgState_Default/6(GeDCC_DCConnSt_enum)  "<GeDCC_DCConnSt_enum>"
  DCChrgState/2(LcDCC_DCChrgCurrRqst_A) -> DCChrgCrntCalc/2(LcDCC_DCChrgCurrRqst_A)
  DCChrgCrntCalc/1(GcDCC_DCChrgCrntRqst_A) -> Unit Delay1/1, GcDCC_DCChrgCrntRqst_A/1
  DCChrgState/1(GeDCC_DCChrgState_enum) -> DCC_GeDCC_DCChrgState_enum/1
  DCC_GeDCC_DCChrgState_enum/1 -> GeDCC_DCChrgState_enum/1, Unit Delay2/1, DCChrgCrntCalc/1(GeDCC_DCChrgState_enum)  "GeDCC_DCChrgState_enum"
  DCChrgState/3(GcDCC_DCChrgVoltRqst_V) -> DCC_GcDCC_DCChrgVoltRqst_V/1
  DCC_GcDCC_DCChrgVoltRqst_V/1 -> GcDCC_DCChrgVoltRqst_V/1  "GcDCC_DCChrgVoltRqst_V"
  DCChrgState/4(GbDCC_DCChrgFinish_flg) -> DCC_GbDCC_DCChrgFinish_flg/1
  DCC_GbDCC_DCChrgFinish_flg/1 -> GbDCC_DCChrgFinish_flg/1  "GbDCC_DCChrgFinish_flg"
  Bus Selector5/1 -> Relational Operator2/1  "<GeDCC_DCChrgState_enum>"
  Constant2/1 -> Relational Operator2/2
  Relational Operator2/1 -> DCChrgState_Default/Enable
  Unit Delay2/1 -> Data Type Conversion1/1
  Constant1/1 -> Relational Operator1/2
  Bus Selector2/1 -> Relational Operator1/1  "<GeDCC_DCChrgState_enum>"
  Relational Operator1/1 -> DCChrgState_Chrg/Enable
  Bus Selector1/1 -> DCChrgState_Chrg/1(GcDCC_DCChrgCrntRqst_A)  "<GcDCC_DCChrgCrntRqst_A>"
  Bus Selector1/2 -> DCChrgState_Chrg/2(GcCDP_MaxCellVolt_mV)  "<GcCDP_MaxCellVolt_mV>"
  Bus Selector1/3 -> DCChrgState_Chrg/3(GeBTM_HeatReq_enum)  "<GeBTM_HeatReq_enum>"
  Bus Selector1/4 -> DCChrgState_Chrg/4(GbDCC_DCChrgPrmt_flg)  "<GbDCC_DCChrgPrmt_flg>"
  Bus Selector1/5 -> DCChrgState_Chrg/5(GeVDP_ChrgRqst_enum)  "<GeVDP_ChrgRqst_enum>"
  Bus Selector3/1 -> DCChrgState_StepChrg/1(GcDCC_DCChrgCrntRqst_A)  "<GcDCC_DCChrgCrntRqst_A>"
  Bus Selector3/2 -> DCChrgState_StepChrg/2(GcCDP_MaxCellVolt_mV)  "<GcCDP_MaxCellVolt_mV>"
  Bus Selector3/3 -> DCChrgState_StepChrg/3(GbDCC_DCChrgPrmt_flg)  "<GbDCC_DCChrgPrmt_flg>"
  Bus Selector3/4 -> DCChrgState_StepChrg/4(GeVDP_ChrgRqst_enum)  "<GeVDP_ChrgRqst_enum>"
  Relational Operator3/1 -> DCChrgState_StepChrg/Enable
  Bus Selector4/1 -> Relational Operator3/1  "<GeDCC_DCChrgState_enum>"
  Constant3/1 -> Relational Operator3/2
  Bus Creator/1 -> Bus Selector4/1, Bus Selector3/1, Bus Selector8/1, Bus Selector9/1, Bus Selector7/1, Bus Selector6/1, Bus Selector1/1, Bus Selector2/1, Bus Selector5/1, Bus Selector/1
  Constant4/1 -> Relational Operator4/2
  Bus Selector6/1 -> Relational Operator4/1  "<GeDCC_DCChrgState_enum>"
  Relational Operator4/1 -> DCChrgState_Stop/Enable
  Bus Selector7/3 -> DCChrgCrntCalc/5(GcVDP_ChrgLdReq_numb)  "<GcVDP_ChrgLdReq_numb>"
  Bus Selector7/4 -> DCChrgCrntCalc/6(GcHDP_PackVolt_V)  "<GcHDP_PackVolt_V>"
  Bus Selector7/5 -> DCChrgCrntCalc/7(GcCDP_MaxCellVolt_mV)  "<GcCDP_MaxCellVolt_mV>"
  DCChrgState_Default/1(LbDCC_ChrgStateDef2Chrg_flg) -> DCChrgState/1(LbDCC_ChrgStateDef2Chrg_flg)
  DCChrgState_Chrg/1(LbDCC_ChrgSt2StepChrg_flg) -> LbDCC_ChrgSt2StepChrg_flg/1, DCChrgState/2(LbDCC_ChrgSt2StepChrg_flg)
  DCChrgState_Chrg/2(LbDCC_ChrgSt2Stop_flg) -> DCChrgState/3(LbDCC_ChrgSt2Stop_flg)
  DCChrgState_Chrg/3(LbDCC_FinishInChrgSt_flg) -> DCChrgState/4(LbDCC_FinishInChrgSt_flg)
  DCChrgState_Chrg/4(GbDCC_DCCrntUnctrolFlt_flg) -> GbDCC_DCCrntUnctrolFlt_flg/1
  DCChrgState_StepChrg/1(LcDCC_StepChrgCrntReq_A) -> DCChrgState/5(LcDCC_StepChrgCrntReq_A)
  DCChrgState_StepChrg/2(LbDCC_StepChrg2Stop_flg) -> DCChrgState/6(LbDCC_StepChrg2Stop_flg)
  DCChrgState_StepChrg/3(LbDCC_FinishInStepChrg_flg) -> DCChrgState/7(LbDCC_FinishInStepChrg_flg)
  DCChrgState_Stop/1(LbDCC_Stop2Default_flg) -> DCChrgState/10(LbDCC_Stop2Default_flg)
  Bus Selector8/2 -> DCChrgState/9(GcSOP_MaxChrgCurr_A)  "<GcSOP_MaxChrgCurr_A>"
  Bus Selector1/6 -> DCChrgState_Chrg/6(GeDCC_DCConnSt_enum)  "<GeDCC_DCConnSt_enum>"
  Bus Selector3/5 -> DCChrgState_StepChrg/5(GeDCC_DCConnSt_enum)  "<GeDCC_DCConnSt_enum>"
  Unit Delay1/1 -> Bus Creator/2  "GcDCC_DCChrgCrntRqst_A"
  Data Type Conversion1/1 -> Bus Creator/1  "GeDCC_DCChrgState_enum"
  Bus Selector7/1 -> DCChrgCrntCalc/3(GeBTM_HeatReq_enum)  "<GeBTM_HeatReq_enum>"
  Bus Selector7/2 -> DCChrgCrntCalc/4(GcGDP_CMLCurMaxOut_A)  "<GcGDP_CMLCurMaxOut_A>"
  Bus Selector8/1 -> DCChrgState/8(GcHDP_PackVolt_V)  "<GcHDP_PackVolt_V>"
  Bus Selector9/1 -> DCChrgState_Stop/1(GeDCC_DCConnSt_enum)  "<GeDCC_DCConnSt_enum>"
  GcUDS_FullChrgCutoffVolt_mV/1 -> Bus Creator/15
  Bus Selector/7 -> DCChrgState_Default/7(GcUDS_FullChrgCutoffVolt_mV)  "<GcUDS_FullChrgCutoffVolt_mV>"
  Bus Selector1/7 -> DCChrgState_Chrg/7(GcUDS_FullChrgCutoffVolt_mV)  "<GcUDS_FullChrgCutoffVolt_mV>"
  Bus Selector3/6 -> DCChrgState_StepChrg/6(GcUDS_FullChrgCutoffVolt_mV)  "<GcUDS_FullChrgCutoffVolt_mV>"
  Bus Selector7/6 -> DCChrgCrntCalc/8(GcUDS_FullChrgCutoffVolt_mV)  "<GcUDS_FullChrgCutoffVolt_mV>"

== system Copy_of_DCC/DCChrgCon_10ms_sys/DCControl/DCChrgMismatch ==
  GeDCC_DCChrgState_enum : Inport
  GbGDP_CMLRecOnce_flg : Inport  Port=2
  GcGDP_CMLChrgrMaxVolt_V : Inport  Port=3
  GcGDP_CMLCurMaxOut_A : Inport  Port=4
  BMSDelay : AIWAYS_Powertrain_BMS_lib/Debounce & Delay/BMSDelay
  Constant : Constant  Value=CcDCC_MaxPackVoltLimt_V
  Constant1 : Constant  Value=CcDCC_DCMaxChrgCurr_A
  Constant2 : Constant  Value=Enum_DCCDCChrgState.Enum_DCCDCChrgState_Default
  Constant3 : Constant  Value=ASWTYPE_TRUE
  Constant4 : Constant  Value=DCC_RUNTIME_MS
  Constant5 : Constant  Value=CcDCC_DCChrgMismatch_ms
  DCC_GbDCC_DCChrgMismatch_flg : AIWAYS_Powertrain_BMS_lib/Signals/OverWrite  OverWrite_Value=CbDCC_DCChrgMismatchOvr_flg  OverWrite_flag=CbDCC_DCChrgMismatchOvrSwt_flg
  Data Type Conversion1 : DataTypeConversion
  Logical Operator : Logic  Operator=OR  AllPortsSameDT=off  OutDataTypeStr=boolean
  Logical Operator1 : Logic  Inputs=3  AllPortsSameDT=off  OutDataTypeStr=boolean
  Relational Operator : RelationalOperator  Operator=<  OutDataTypeStr=boolean
  Relational Operator1 : RelationalOperator  Operator=<  OutDataTypeStr=boolean
  Relational Operator2 : RelationalOperator  Operator===  OutDataTypeStr=boolean
  Relational Operator3 : RelationalOperator  Operator===  OutDataTypeStr=boolean
  GbDCC_DCChrgMismatch_flg : Outport
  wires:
  GcGDP_CMLChrgrMaxVolt_V/1 -> Relational Operator/1
  Constant/1 -> Relational Operator/2
  GcGDP_CMLCurMaxOut_A/1 -> Relational Operator1/1
  Constant1/1 -> Relational Operator1/2
  Relational Operator/1 -> Logical Operator/1
  Relational Operator1/1 -> Logical Operator/2
  GbGDP_CMLRecOnce_flg/1 -> Relational Operator3/1
  Constant3/1 -> Relational Operator3/2
  Logical Operator1/1 -> BMSDelay/1  "LbDCC_DCChrgMismatch_flg"
  Constant2/1 -> Relational Operator2/2
  GeDCC_DCChrgState_enum/1 -> Data Type Conversion1/1
  Relational Operator2/1 -> Logical Operator1/1
  Relational Operator3/1 -> Logical Operator1/2
  Logical Operator/1 -> Logical Operator1/3
  Data Type Conversion1/1 -> Relational Operator2/1
  Constant5/1 -> BMSDelay/3
  Constant4/1 -> BMSDelay/2
  BMSDelay/1 -> DCC_GbDCC_DCChrgMismatch_flg/1
  DCC_GbDCC_DCChrgMismatch_flg/1 -> GbDCC_DCChrgMismatch_flg/1  "GbDCC_DCChrgMismatch_flg"

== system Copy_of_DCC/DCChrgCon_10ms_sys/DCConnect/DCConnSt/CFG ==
  GbGDP_CMLRecOnce_flg : Inport
  GbDCC_DCChrgPrmt_flg : Inport  Port=2
  Enable : EnablePort  StatesWhenEnabling=reset
  Constant1 : Constant  Value=DCC_RUNTIME_MS
  Constant2 : Constant  Value=ASWTYPE_TRUE
  Constant5 : Constant  Value=CcDCC_DCChrgPermitCfg_ms
  Constant6 : Constant  Value=ASWTYPE_FALSE
  Delay1 : AIWAYS_Powertrain_BMS_lib/Debounce & Delay/BMSDelay
  Logical Operator1 : Logic  AllPortsSameDT=off  OutDataTypeStr=boolean
  Relational Operator1 : RelationalOperator  Operator===  OutDataTypeStr=boolean
  Relational Operator2 : RelationalOperator  Operator===  OutDataTypeStr=boolean
  LbDCC_DCCFG2ChrgFinish_flg : Outport
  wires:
  Constant1/1 -> Delay1/2
  Constant5/1 -> Delay1/3
  Logical Operator1/1 -> Delay1/1
  Constant6/1 -> Relational Operator1/2
  GbDCC_DCChrgPrmt_flg/1 -> Relational Operator1/1
  Delay1/1 -> LbDCC_DCCFG2ChrgFinish_flg/1  "LbDCC_DCCFG2ChrgFinish_flg"
  Relational Operator1/1 -> Logical Operator1/2
  Constant2/1 -> Relational Operator2/2
  Relational Operator2/1 -> Logical Operator1/1
  GbGDP_CMLRecOnce_flg/1 -> Relational Operator2/1

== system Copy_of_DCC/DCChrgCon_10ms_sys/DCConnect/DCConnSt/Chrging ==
  GbGDP_CSTRecOnce_flg : Inport
  GbDCC_DCChrgPrmt_flg : Inport  Port=2
  GbDCC_DCChrgFinish_flg : Inport  Port=3
  Enable : EnablePort  StatesWhenEnabling=reset
  Constant1 : Constant  Value=DCC_RUNTIME_MS
  Constant2 : Constant  Value=ASWTYPE_TRUE
  Constant3 : Constant  Value=DCC_RUNTIME_MS
  Constant4 : Constant  Value=CcDCC_DCChrgPrmtStop_ms
  Constant5 : Constant  Value=CcDCC_DCChrgStop_ms
  Constant6 : Constant  Value=ASWTYPE_FALSE
  Delay1 : AIWAYS_Powertrain_BMS_lib/Debounce & Delay/BMSDelay
  Delay2 : AIWAYS_Powertrain_BMS_lib/Debounce & Delay/BMSDelay
  Logical Operator : Logic  Operator=OR  Inputs=3  AllPortsSameDT=off  OutDataTypeStr=boolean
  Relational Operator1 : RelationalOperator  Operator===  OutDataTypeStr=boolean
  Relational Operator2 : RelationalOperator  Operator===  OutDataTypeStr=boolean
  LbDCC_DCChrging2ChrgFin_flg : Outport
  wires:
  Logical Operator/1 -> LbDCC_DCChrging2ChrgFin_flg/1  "LbDCC_DCChrging2ChrgFin_flg"
  GbDCC_DCChrgPrmt_flg/1 -> Relational Operator1/1
  Constant6/1 -> Relational Operator1/2
  GbDCC_DCChrgFinish_flg/1 -> Delay1/1
  Constant5/1 -> Delay1/3
  Delay1/1 -> Logical Operator/3
  Constant1/1 -> Delay1/2
  Constant2/1 -> Relational Operator2/2
  GbGDP_CSTRecOnce_flg/1 -> Relational Operator2/1
  Relational Operator2/1 -> Logical Operator/1
  Relational Operator1/1 -> Delay2/1
  Delay2/1 -> Logical Operator/2
  Constant3/1 -> Delay2/2
  Constant4/1 -> Delay2/3

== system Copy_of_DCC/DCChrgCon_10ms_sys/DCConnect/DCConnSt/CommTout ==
  GeCTC_CtrCtlConnMode_enum : Inport
  GbGDP_CHMRecOnce_flg : Inport  Port=2
  GbGDP_CRMRecOnce_flg : Inport  Port=3
  GbLDP_DC12VSply_flg : Inport  Port=4
  Enable : EnablePort  StatesWhenEnabling=reset
  Constant : Constant  Value=Enum_CTCCtrCtlConnMode.Enum_CTCCtrCtlConnMode_DCChrg
  Constant{1,5..7} (4 alike) : Constant  Value=ASWTYPE_TRUE
  Constant2 : Constant  Value=DCC_RUNTIME_MS
  Constant3 : Constant  Value=CcDCC_ToutDelay_ms
  Data Type Conversion1 : DataTypeConversion
  Delay : AIWAYS_Powertrain_BMS_lib/Debounce & Delay/BMSDelay
  Logical Operator : Logic  Inputs=3  AllPortsSameDT=off  OutDataTypeStr=boolean
  Logical Operator1 : Logic  Operator=OR  Inputs=3  AllPortsSameDT=off  OutDataTypeStr=boolean
  Relational Operator1 : RelationalOperator  Operator===  OutDataTypeStr=boolean
  Relational Operator2 : RelationalOperator  Operator===  OutDataTypeStr=boolean
  Relational Operator4 : RelationalOperator  Operator=~=  OutDataTypeStr=boolean
  Relational Operator6 : RelationalOperator  Operator===  OutDataTypeStr=boolean
  LbDCC_DCCommTout2Default_flg : Outport
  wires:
  Logical Operator/1 -> LbDCC_DCCommTout2Default_flg/1  "LbDCC_DCCommTout2Default_flg"
  Logical Operator1/1 -> Logical Operator/2
  Relational Operator4/1 -> Logical Operator/1
  Constant/1 -> Relational Operator4/2
  GeCTC_CtrCtlConnMode_enum/1 -> Data Type Conversion1/1
  GbLDP_DC12VSply_flg/1 -> Relational Operator6/1
  Constant5/1 -> Relational Operator6/2
  Relational Operator6/1 -> Logical Operator1/3
  Constant3/1 -> Delay/3
  Constant1/1 -> Delay/1
  Constant2/1 -> Delay/2
  Delay/1 -> Logical Operator/3
  Constant6/1 -> Relational Operator1/2
  GbGDP_CRMRecOnce_flg/1 -> Relational Operator1/1
  Relational Operator1/1 -> Logical Operator1/2
  Constant7/1 -> Relational Operator2/2
  GbGDP_CHMRecOnce_flg/1 -> Relational Operator2/1
  Relational Operator2/1 -> Logical Operator1/1
  Data Type Conversion1/1 -> Relational Operator4/1

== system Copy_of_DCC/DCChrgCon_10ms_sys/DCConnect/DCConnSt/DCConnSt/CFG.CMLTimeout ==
  GbGDP_CMLRecOnce_flg : Inport  OutDataTypeStr=boolean
  CMLTimeout : TriggerPort  TriggerType=function-call  VariantControl=(inherit)  StatesWhenEnabling=reset
  Constant : Constant  Value=ASWTYPE_TRUE
  Constant2 : Constant  Value=DCC_RUNTIME_MS
  Constant3 : Constant  Value=CcDCC_CMLTout_ms
  Constant4 : Constant  Value=ASWTYPE_FALSE
  Delay : AIWAYS_Powertrain_BMS_lib/Debounce & Delay/BMSDelay
  Logical Operator : Logic  AllPortsSameDT=off  OutDataTypeStr=boolean
  Relational Operator : RelationalOperator  Operator===  OutDataTypeStr=boolean
  GbDCC_CMLTout_flg : Outport  OutDataTypeStr=boolean
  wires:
  GbGDP_CMLRecOnce_flg/1 -> Relational Operator/1
  Constant3/1 -> Delay/3
  Relational Operator/1 -> Logical Operator/1
  Constant2/1 -> Delay/2
  Delay/1 -> Logical Operator/2
  Constant4/1 -> Relational Operator/2
  Constant/1 -> Delay/1
  Logical Operator/1 -> GbDCC_CMLTout_flg/1

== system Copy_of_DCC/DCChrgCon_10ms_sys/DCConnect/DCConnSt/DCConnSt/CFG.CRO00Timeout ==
  GbGDP_CRORecOnce_flg : Inport  OutDataTypeStr=boolean
  GbDCC_BROMsgCmd_flg : Inport  Port=2  OutDataTypeStr=boolean
  GcGDP_CROChrgrRdy_numb : Inport  Port=3  OutDataTypeStr=uint8
  GcDCS_2829Da_numb : Inport  Port=4  OutDataTypeStr=uint8
  CROTimeout : TriggerPort  TriggerType=function-call  VariantControl=(inherit)  StatesWhenEnabling=reset
  Constant1 : Constant  Value=DCC_RUNTIME_MS
  Constant11 : Constant  Value=DCC_CONST0_NUMB
  Constant2 : Constant  Value=ASWTYPE_FALSE
  Constant5 : Constant  Value=CcDCC_CROTout_ms
  Constant6 : Constant  Value=ASWTYPE_FALSE
  Constant7 : Constant  Value=DCC_CONST170_NUMB
  Delay1 : AIWAYS_Powertrain_BMS_lib/Debounce & Delay/BMSDelay
  Logical Operator : Logic  AllPortsSameDT=off  OutDataTypeStr=boolean
  Logical Operator1 : Logic  Inputs=3  AllPortsSameDT=off  OutDataTypeStr=boolean
  Logical Operator3 : Logic  Operator=OR  AllPortsSameDT=off  OutDataTypeStr=boolean
  Logical Operator4 : Logic  Operator=OR  AllPortsSameDT=off  OutDataTypeStr=boolean
  Relational Operator{1..3,5} (4 alike) : RelationalOperator  Operator===  OutDataTypeStr=boolean
  Unit Delay : UnitDelay  SampleTime=-1  StateName=StateName
  GbDCC_CROTout_flg : Outport  OutDataTypeStr=boolean
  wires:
  GcDCS_2829Da_numb/1 -> Relational Operator2/1
  GbGDP_CRORecOnce_flg/1 -> Logical Operator/2, Relational Operator1/1
  Logical Operator1/1 -> GbDCC_CROTout_flg/1
  Relational Operator2/1 -> Delay1/1
  Constant1/1 -> Delay1/2
  Constant6/1 -> Relational Operator1/2
  Constant5/1 -> Delay1/3
  Constant7/1 -> Relational Operator2/2
  Constant11/1 -> Relational Operator5/2
  GcGDP_CROChrgrRdy_numb/1 -> Relational Operator5/1
  Constant2/1 -> Relational Operator3/2
  Relational Operator3/1 -> Logical Operator3/1
  Relational Operator1/1 -> Logical Operator3/2
  GbDCC_BROMsgCmd_flg/1 -> Logical Operator1/2
  Delay1/1 -> Logical Operator1/3
  Logical Operator3/1 -> Logical Operator1/1
  Logical Operator4/1 -> Relational Operator3/1, Unit Delay/1
  Relational Operator5/1 -> Logical Operator/1
  Logical Operator/1 -> Logical Operator4/2
  Unit Delay/1 -> Logical Operator4/1
